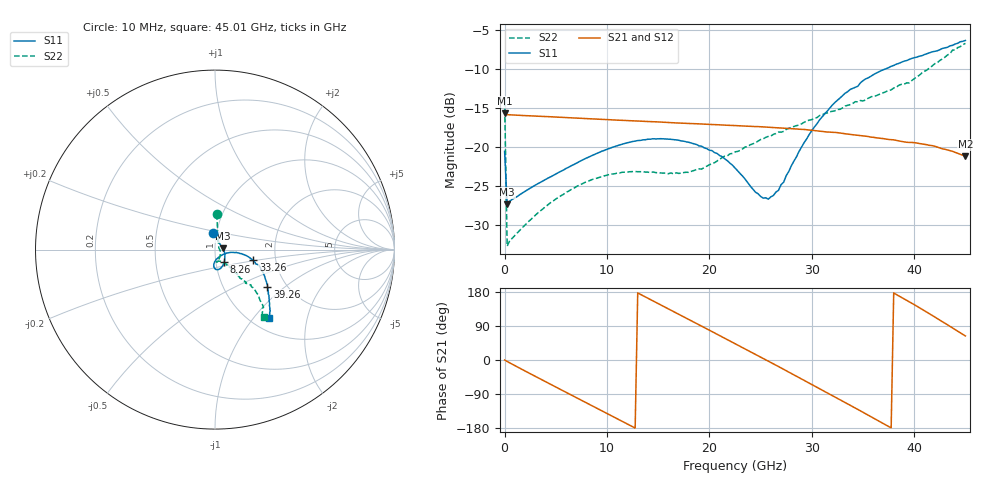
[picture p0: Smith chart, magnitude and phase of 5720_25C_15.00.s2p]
! Device:  ADRF5720
! Description: 0.5dB LSB GaAs MMIC 6-bit Digital Attenuator
! Frequency:  0.000009 -  40 GHz
! Ports:
!	RF1	= Port 1
!	RF2	= Port 2
! Vdd:  3.3 Volt
! Vss:  -3.3 Volt
! Control:  0/3.3 Volt
! State:  15.00 dB attenuation
! Data:  The device was measured using G-S-G Probes on a matrix board.
!  Data was collected using an calibrated 4 port network analyzer.
!  The reference plane for this measurement is at the launchers.
! Note:  Analog Devices supplies this data as a sample of measured data
!  for this product.  Your particular data for this product may vary.
!  Data was taken at 25 degrees C.
!  Analog Devices reserves the right to change this data at anytime.
# GHZ S DB R 45.0
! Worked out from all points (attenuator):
!   181 points, 10 MHz to 45.01 GHz, reference 45 ohm
!   highest |S21| = -15.67 dB at 10 MHz (marker M1); lowest = -21.2 dB at 45.01 GHz (marker M2)
!   lowest |S11| = -27.4 dB at 260 MHz (marker M3), VSWR 1.09, Z = 48.9 + j0.81 ohm
!   |S11| at or under -10 dB: start of sweep to 37.14 GHz
!   |S22| runs from -32.8 to -6.7 dB; largest |S21 - S12| = 0.0002
!   S11 on the Smith chart (normalised r, x): 10 MHz: 0.96, +0.18; 8.26 GHz: 1.10, -0.15; 33.26 GHz: 1.53, -0.19; 39.26 GHz: 1.60, -0.77; 45.01 GHz: 1.21, -1.20
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0.01  -20.59 96.8  -15.67 -0.1  -15.67 -0.1  -14.05 87.5
0.26  -27.38 11.1  -15.86 -3.9  -15.86 -3.9  -32.79 20.1
1.26  -26.38 -2.9  -15.92 -18.4  -15.93 -18.4  -31.04 -7.6
4.26  -24.02 -29.0  -16.11 -60.8  -16.12 -60.8  -27.44 -46.7
7.76  -21.60 -50.6  -16.34 -109.8  -16.34 -109.8  -24.64 -68.8
8.26  -21.30 -53.2  -16.38 -116.8  -16.38 -116.8  -24.38 -70.6
11.76  -19.56 -69.4  -16.60 -165.6  -16.61 -165.6  -23.26 -80.3
15.26  -18.95 -82.5  -16.81 145.3  -16.81 145.3  -23.36 -80.2
19.26  -19.93 -92.7  -17.06 89.2  -17.06 89.2  -22.86 -65.0
21.26  -21.27 -94.2  -17.18 61.0  -17.19 61.0  -21.38 -58.1
22.76  -23.07 -92.3  -17.28 39.8  -17.28 39.8  -20.59 -54.2
24.51  -25.84 -75.3  -17.39 15.1  -17.39 15.1  -19.48 -52.1
25.76  -26.74 -51.7  -17.47 -2.9  -17.47 -2.9  -18.66 -51.2
27.26  -24.56 -21.9  -17.58 -24.6  -17.58 -24.6  -18.01 -49.3
28.76  -20.60 -9.3  -17.73 -46.2  -17.73 -46.1  -17.19 -49.3
30.26  -17.45 -8.0  -17.90 -68.2  -17.90 -68.1  -16.31 -48.6
33.26  -13.10 -15.7  -18.33 -112.2  -18.33 -112.2  -14.75 -47.8
35.51  -11.12 -23.1  -18.67 -145.6  -18.67 -145.6  -13.74 -48.0
37.76  -9.63 -30.9  -19.07 -179.2  -19.08 -179.2  -12.67 -46.7
39.26  -8.90 -35.5  -19.41 157.9  -19.41 158.0  -11.77 -47.0
42.26  -7.63 -43.5  -20.02 109.1  -20.02 109.2  -9.16 -46.4
45.01  -6.30 -51.5  -21.21 63.5  -21.21 63.6  -6.68 -54.3
